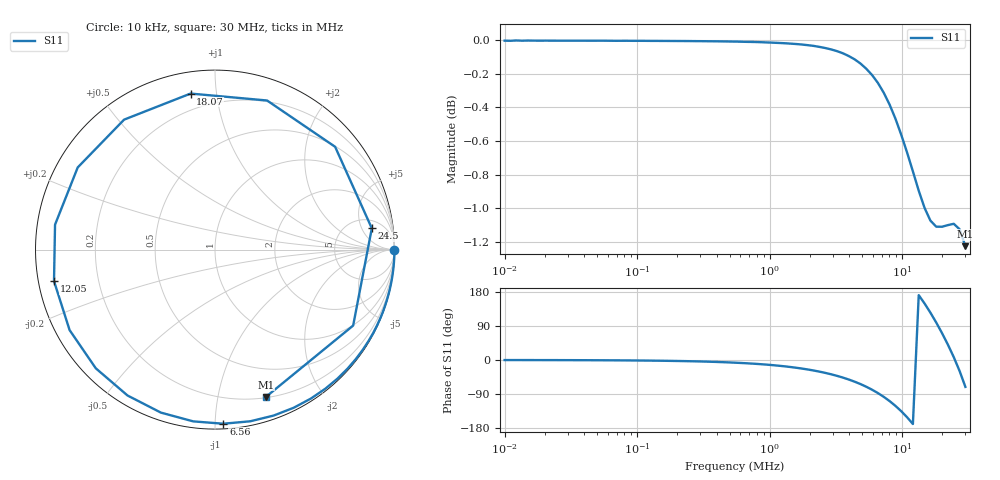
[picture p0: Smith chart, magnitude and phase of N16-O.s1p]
! ListType=Log
!!2-Port #16 Magnet Open
# MHz S RI R 50
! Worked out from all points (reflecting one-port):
!   80 points, 10 kHz to 30 MHz, reference 50 ohm
!   lowest |S11| = -1.2 dB at 30 MHz (marker M1), VSWR 14.18, Z = 10.4 - j69.2 ohm
!   phase of S11 starts at -0 deg and turns -431 deg over the sweep
!   S11 on the Smith chart (normalised r, x): 10 kHz: open; 6.56 MHz: 0.03, -1.05; 12.05 MHz: 0.05, -0.10; 18.07 MHz: 0.11, +0.85; 24.5 MHz: 7, +8; 30 MHz: 0.21, -1.38
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0.01  0.9998 -0.00235
0.0275513  0.9998 -0.00628
0.0759074  0.9996 -0.0172
0.2091346  0.9985 -0.0472
0.5761927  0.9908 -0.1293
0.9563981  0.9756 -0.2132
1.587485  0.9345 -0.3489
2.151554  0.8813 -0.4645
2.916049  0.7855 -0.6088
3.571274  0.6832 -0.7181
4.373726  0.5354 -0.8293
5.356486  0.3272 -0.9246
6.560068  0.0465 -0.9701
7.259765  -0.1211 -0.9571
8.034091  -0.3017 -0.9081
8.891007  -0.4875 -0.8127
9.839321  -0.664 -0.6615
10.88878  -0.8102 -0.4483
12.05018  -0.897 -0.1756
13.33545  -0.8912 0.139
14.75781  -0.7649 0.4577
16.33188  -0.5065 0.7241
18.07383  -0.1359 0.8694
20.00159  0.2902 0.8307
22.13496  0.6693 0.5727
24.49587  0.8737 0.1186
27.1086  0.7697 -0.4233
30  0.2837 -0.8206
